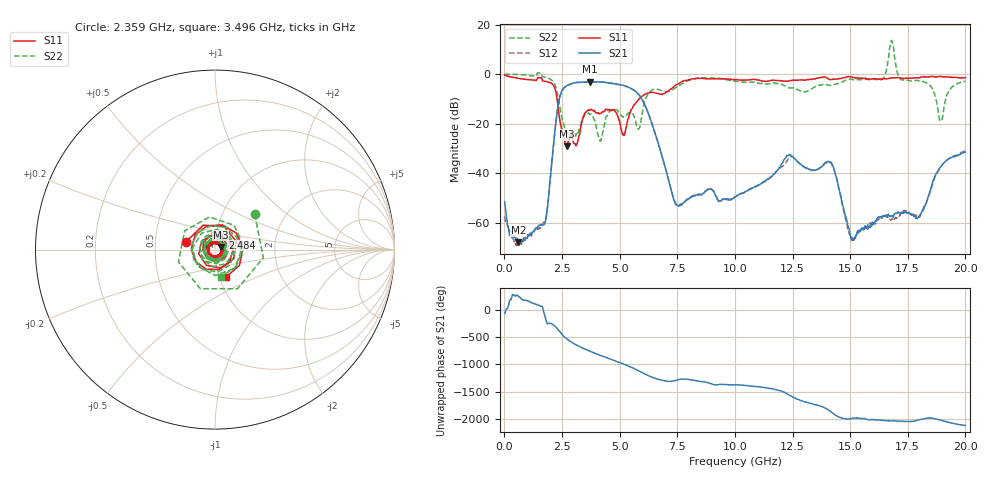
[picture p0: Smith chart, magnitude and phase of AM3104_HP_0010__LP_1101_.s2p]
!Created with skrf (http://scikit-rf.org).
# Hz S RI R 50.0
!freq ReS11 ImS11 ReS21 ImS21 ReS12 ImS12 ReS22 ImS22
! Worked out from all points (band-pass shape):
!   1601 points, 10 MHz to 20 GHz, reference 50 ohm
!   highest |S21| = -3.07 dB at 3.696 GHz (marker M1); lowest = -67.8 dB at 609.7 MHz (marker M2)
!   |S21| within 3 dB of the highest: 2.541 GHz to 5.557 GHz (3.017 GHz wide, 74.5 % of centre)
!   lowest |S11| = -29.1 dB at 2.709 GHz (marker M3), VSWR 1.07, Z = 53.2 + j1.64 ohm
!   |S11| at or under -10 dB: 2.285 GHz to 5.844 GHz (3.559 GHz wide, 87.6 % of centre)
!   |S22| runs from -27.1 to 13.6 dB; largest |S21 - S12| = 0.07
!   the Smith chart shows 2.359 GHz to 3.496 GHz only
!   S11 on the Smith chart (normalised r, x): 2.359 GHz: 0.72, +0.07; 2.484 GHz: 1.08, +0.14; 3.496 GHz: 1.08, -0.34
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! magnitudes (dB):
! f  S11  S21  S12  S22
! 10 MHz  -0.4  -51.5  -57.4  0.0
! 609.7 MHz  -1.7  -67.8  -68.7  -0.1
! 1.759 GHz  -2.8  -60.2  -59.3  -1.2
! 2.359 GHz  -15.6  -11.1  -11.2  -10.6
! 2.484 GHz  -22.1  -7.0  -7.0  -16.8
! 2.709 GHz  -29.1  -4.6  -4.6  -23.5
! 3.346 GHz  -20.0  -3.2  -3.3  -19.1
! 3.496 GHz  -15.7  -3.2  -3.2  -16.2
! 3.696 GHz  -14.6  -3.1  -3.2  -16.2
! 4.158 GHz  -15.9  -3.1  -3.2  -27.1
! 5.17 GHz  -24.2  -4.5  -4.6  -17.1
! 5.72 GHz  -11.4  -7.2  -7.2  -20.2
! 6.682 GHz  -7.9  -28.1  -28.1  -6.2
! 7.506 GHz  -4.1  -53.0  -53.0  -5.0
! 10.01 GHz  -2.3  -49.7  -49.7  -2.9
! 13.34 GHz  -2.1  -38.8  -38.8  -5.9
! 14.22 GHz  -2.2  -36.5  -36.7  -4.4
! 15.1 GHz  -1.3  -67.0  -66.2  -2.2
! 16.68 GHz  -1.7  -56.9  -58.3  7.3
! 17.95 GHz  -1.4  -57.8  -57.4  -2.6
! 18.93 GHz  -0.8  -37.4  -37.5  -18.9
! 20 GHz  -1.4  -31.5  -30.8  -2.8
